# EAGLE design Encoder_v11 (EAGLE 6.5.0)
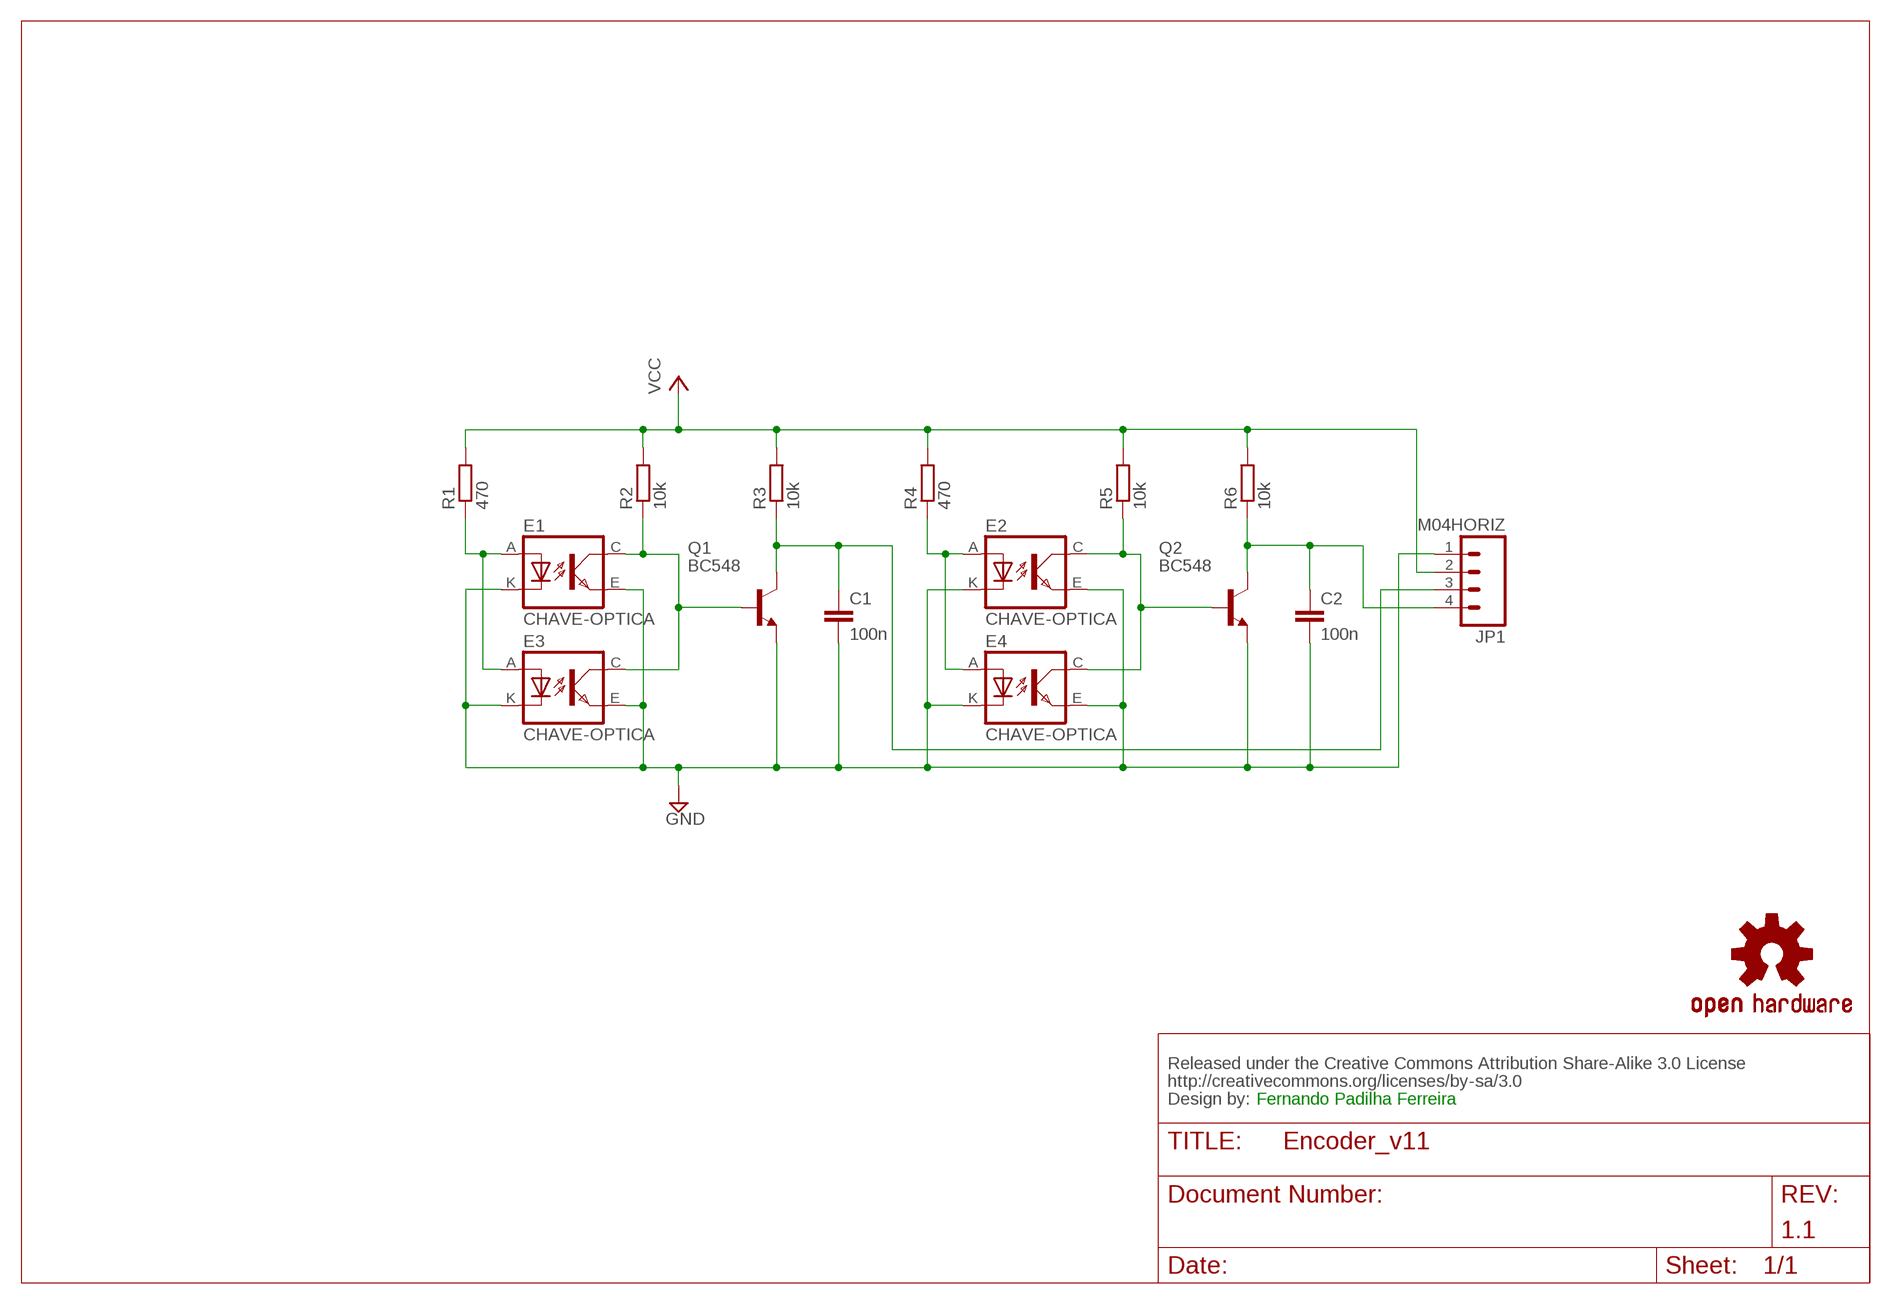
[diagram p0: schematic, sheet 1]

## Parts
C1  100n  C5/2.5  [C5B2.5]
C2  100n  C5/2.5  [C5B2.5]
CC_TEXT1  CREATIVE_COMMONS  [CREATIVE_COMMONS]
E1  CHAVE-OPTICA  [PHCT103]
E2  CHAVE-OPTICA  [PHCT103]
E3  CHAVE-OPTICA  [PHCT103]
E4  CHAVE-OPTICA  [PHCT103]
JP1  M04HORIZ  [1X04_HORIZ]
LOGO1  OSHW-LOGOL  [OSHW-LOGO-L]
Q1  BC548  [TO92-EBC]
Q2  BC548  [TO92-EBC]
R1  470  R-EU_0207/10  [0207/10]
R2  10k  R-EU_0207/10  [0207/10]
R3  10k  R-EU_0207/10  [0207/10]
R4  470  R-EU_0207/10  [0207/10]
R5  10k  R-EU_0207/10  [0207/10]
R6  10k  R-EU_0207/10  [0207/10]

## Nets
GND: C1.2 C2.2 E1.E(EMIT) E1.K E2.E(EMIT) E2.K E3.E(EMIT) E3.K E4.E(EMIT) E4.K JP1.1 Q1.E Q2.E
N$1: E1.C(COL) E3.C(COL) Q1.B R2.1
N$2: E2.C(COL) E4.C(COL) Q2.B R5.1
N$3: E2.A E4.A R4.1
N$4: E1.A E3.A R1.1
N$5: C1.1 JP1.3 Q1.C R3.1
N$6: C2.1 JP1.4 Q2.C R6.1
VCC: JP1.2 R1.2 R2.2 R3.2 R4.2 R5.2 R6.2

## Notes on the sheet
- Fernando Padilha Ferreira
- 1.1

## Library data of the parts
C1 C2 = capacitor-wima:C: CAPACITOR
CC_TEXT1 = SparkFun-Aesthetics:CREATIVE_COMMONS: Creative Commons License summary
E1-E4 = FernandoLib:CHAVE-OPTICA
JP1 = FernandoLib:M04
LOGO1 = SparkFun-Aesthetics:OSHW-LOGO: Open Source Hardware Logo This logo indicates the piece of hardware it is found on incorporates a OSHW license and/or adheres to the definition of open source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
Q1 Q2 = transistor-npn:BC548*: NPN Transistor
R1-R6 = resistor:R-EU_: RESISTOR, European symbol

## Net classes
0 default: width 0.305 mm

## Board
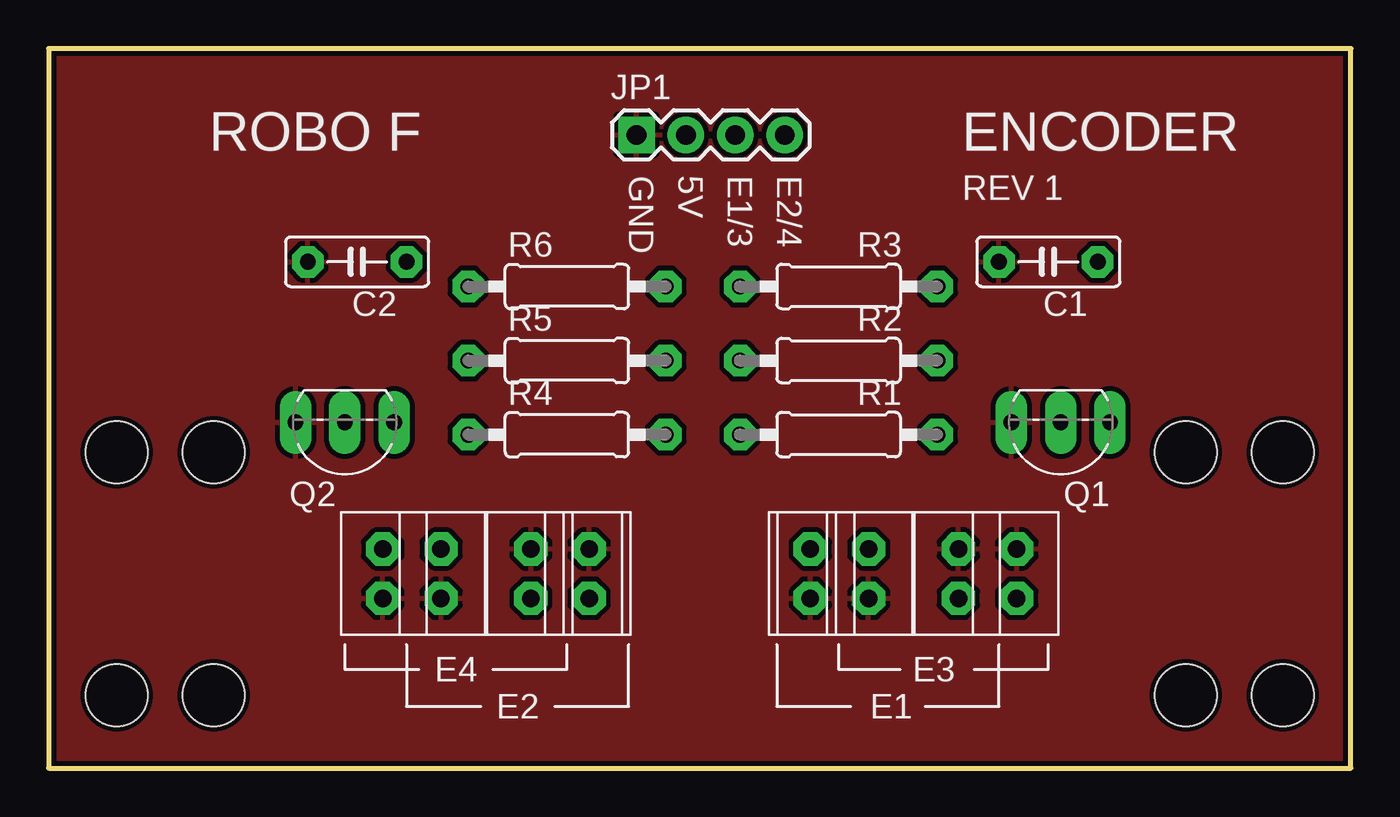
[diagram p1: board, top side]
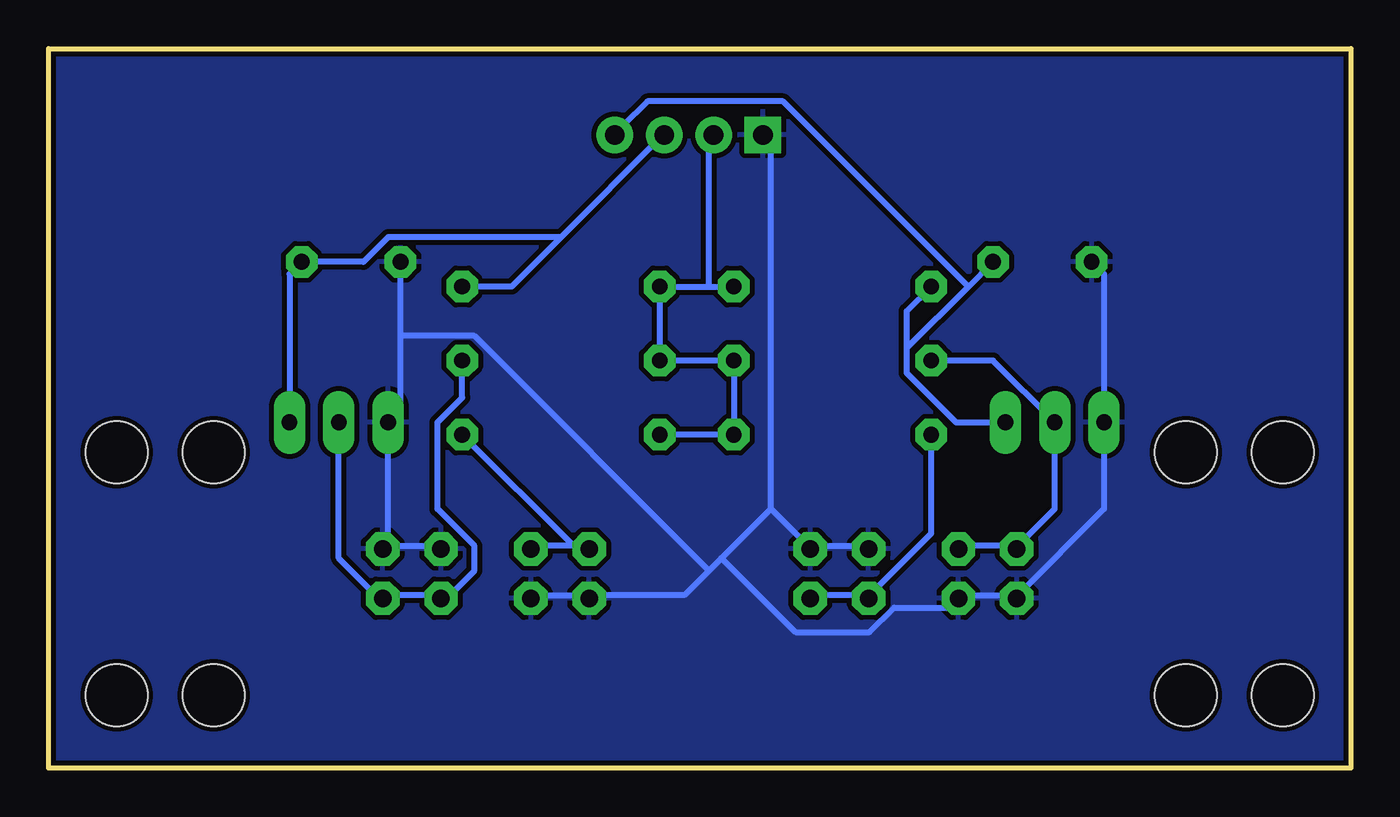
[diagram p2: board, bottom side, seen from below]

Size 67 x 37 mm. Coordinates in mm from the lower left corner, seen from the top.
Outline: 0,0 67,0 67,37 0,37 0,0
Copper layers (1*16): Top 0.035mm / dielectric 1.5mm / Bottom 0.035mm
Design rules "peteco *": minimum track width 12mil, minimum drill 19mil, track to track 10mil, track to pad 10mil, pad to pad 10mil, via to via 10mil, smd to smd 0mil, copper to edge 10mil, drill to drill 8mil, minimum pad ring 16mil, minimum via ring 8mil, stop-mask expansion 4mil, vias tented up to drill 0mil, thermal gap 10mil
Holes 3.2 mm at 3.5,3.75 3.5,16.25 63.5,3.75 63.5,16.25 8.5,16.25 58.5,16.25 8.5,3.75 58.5,3.75

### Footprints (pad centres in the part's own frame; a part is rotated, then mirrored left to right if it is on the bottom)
C5B2.5 = drill 0.813 pad 1.6 octagon: 1 -2.54,0; 2 2.54,0
PHCT103 = drill 0.9 pad 1.676 octagon: A -3.81,1.27; C 3.81,-1.27; E 3.81,1.27; K -3.81,-1.27
1X04_HORIZ = drill 1.016 pad 1.88 square: 1 0,0 | drill 1.016 pad 1.88: 2 2.54,0; 3 5.08,0; 4 7.62,0
TO92-EBC = drill 0.813 long: B 0,-1.27; C -2.54,-1.27; E 2.54,-1.27
0207/10 = drill 0.813 octagon: 1 -5.08,0; 2 5.08,0

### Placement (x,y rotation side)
C1  51.44,26.04 180 top
C2  15.88,26.04 180 top
CC_TEXT1  not placed on the board
E1  43,10 0 top
E2  24,10 180 top
E3  46,10 0 top
E4  21,10 180 top
JP1  30.25,32.56 0 top
LOGO1  not placed on the board
Q1  52.07,16.51 180 top
Q2  15.24,16.51 180 top
R1  40.64,17.14 180 top
R2  40.64,20.95 180 top
R3  40.64,24.77 180 top
R4  26.67,17.14 0 top
R5  26.67,20.95 0 top
R6  26.67,24.77 0 top

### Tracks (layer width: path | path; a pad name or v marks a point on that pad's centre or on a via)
GND
  Bottom 0.305: C2.2 12.7,25.4 Q2.E 12.7,13.34 17.14,8.89 E4.E 17.78,8.89 19.68,8.89 E2.E 20.32,8.26 23.5,8.26 24.77,6.99 28.57,6.99 32.38,10.79 | 49.53,11.43 Q1.E 48.9,18.41 48.9,22.23 | 48.9,22.23 C1.2 | 49.53,11.43 46.99,11.43 E1.E | 49.53,11.43 E3.E | E3.K 41.91,8.89 39.37,8.89 E1.K 38.73,8.89 34.29,8.89 33.02,10.16 | E4.K 25.4,11.43 27.3,11.43 E2.K 27.94,11.43 29.84,13.34 | 29.84,13.34 29.84,32.38 JP1.1 | 29.84,13.34 32.38,10.79 | 32.38,10.79 33.02,10.16 | 48.9,22.23 45.09,22.23 33.02,10.16
  pour Bottom: 0,36.83 67.31,36.83 67.31,0 0,0
  pour Top: 0,36.83 67.31,36.83 67.31,0 0,0
N$1
  Bottom 0.305: Q1.B 52.07,10.79 50.16,8.89 E3.C 49.53,8.89 46.99,8.89 E1.C 46.35,8.89 45.09,10.16 45.09,11.43 46.99,13.34 46.99,17.78 45.72,19.05 R2.1
N$2
  Bottom 0.305: R5.1 18.41,20.95 Q2.B 15.24,13.34 17.14,11.43 E4.C 17.78,11.43 19.68,11.43 E2.C
N$3
  Bottom 0.305: R4.1 21.59,12.06 24.77,8.89 E4.A 25.4,8.89 27.3,8.89 E2.A
N$4
  Bottom 0.305: 40.01,11.43 39.37,10.79 E1.A 40.01,11.43 | 40.01,11.43 R1.1 | 40.01,11.43 41.91,11.43 E3.A
N$5
  Bottom 0.305: Q1.C 54.61,25.4 C1.1 50.8,26.04 49.53,27.3 40.64,27.3 | R3.1 43.18,24.77 40.64,27.3 | 40.64,27.3 35.56,32.38 JP1.3
N$6
  Bottom 0.305: Q2.C 20.32,17.78 22.86,20.32 22.86,21.59 | 22.86,21.59 22.86,23.5 R6.1 | 22.86,21.59 19.68,24.77 | 19.68,24.77 C2.1 | 19.68,24.77 29.21,34.29 36.2,34.29 37.47,33.02 JP1.4
VCC
  Bottom 0.305: R1.2 R4.2 R5.2 R2.2 R3.2 33.02,24.77 | 33.02,24.77 R6.2 | 33.02,24.77 33.02,32.38 JP1.2

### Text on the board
tPlace: ROBO F | ENCODER | GND | 5V | E1/3 | E2/4 | REV 1
tValues: PHCT103 | PHCT103
tDocu: Fernando Padilha Ferreira

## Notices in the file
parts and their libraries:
SparkFun-Aesthetics: Licensing: CC v3.0 Share-Alike You are welcome to use this library for commercial purposes.
SparkFun-Aesthetics: Released under the Creative Commons Attribution Share-Alike 3.0 License
SparkFun-Aesthetics: http://creativecommons.org/licenses/by-sa/3.0
